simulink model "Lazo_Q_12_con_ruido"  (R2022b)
settings: Solver=ode4  StartTime=0.0  StopTime=0.2  FixedStep=1e-6  RelTol=1e-3
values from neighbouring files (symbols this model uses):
  Delta_v_d_1 = P_Delta_v_d_1*v_d_12    [IP_Lazo_Q_12.m]    (also in LQR_Con_Integral.m = 8; Modal_Integral.m = 8)
  Delta_v_d_2 = P_Delta_v_d_2*v_d_12    [IP_Lazo_Q_12.m]    (also in IP_Lazo_P_2.m = P_Delta_v_d_2*v_d_2)
  I_Delta_v_d_1 = 0.15    [IP_Lazo_Q_12.m]
  I_Delta_v_d_2 = 0.15    [IP_Lazo_Q_12.m]    (also in IP_Lazo_P_2.m)
  Ki_Q = ((3*v_d_12*Kp_Q-2)/(3*v_d_12*tau))    [IP_Lazo_Q_12.m]    (also in Sistema_control_no_lineal_LQR.m = ((3*v_d_1*Kp_Q-2)/(3*v_d_1*tau_Q)); Sistema_control_no_lineal_Modal.m = ((3*v_d_1*Kp_Q-2)/(3*v_d_1*tau_Q)))
  Kp_Q = 1    [IP_Lazo_Q_12.m]    (also in Sistema_control_no_lineal_LQR.m = 0.0002; Sistema_control_no_lineal_Modal.m = 0.0002)
  lim_i_q_1_lower = -576.70686    [IP_Lazo_Q_12.m]    (also in Sistema_control_no_lineal_LQR.m; Sistema_control_no_lineal_Modal.m)
  lim_i_q_1_upper = 393.72177    [IP_Lazo_Q_12.m]    (also in Sistema_control_no_lineal_LQR.m; Sistema_control_no_lineal_Modal.m)
  Q_1_1 = 0    [IP_Lazo_Q_12.m]    (also in Sistema_control_no_lineal_LQR.m; Sistema_control_no_lineal_Modal.m)
  Q_1_2 = -2500    [IP_Lazo_Q_12.m]    (also in Sistema_control_no_lineal_LQR.m = 0; Sistema_control_no_lineal_Modal.m = 0)
  Q_2_1 = -3000    [IP_Lazo_Q_12.m]    (also in Sistema_control_no_lineal_LQR.m = 0; Sistema_control_no_lineal_Modal.m = 0)
  Q_2_2 = 1000    [IP_Lazo_Q_12.m]    (also in Sistema_control_no_lineal_LQR.m = 0; Sistema_control_no_lineal_Modal.m = 0)
  v_d_12 = 100*sqrt(2)    [IP_Lazo_Q_12.m]
  V_R_Q_1 = D_R_Q_1^2    (= 0.0009)    [IP_Lazo_Q_12.m]
  V_R_Q_2 = D_R_Q_2^2    (= 0.0009)    [IP_Lazo_Q_12.m]

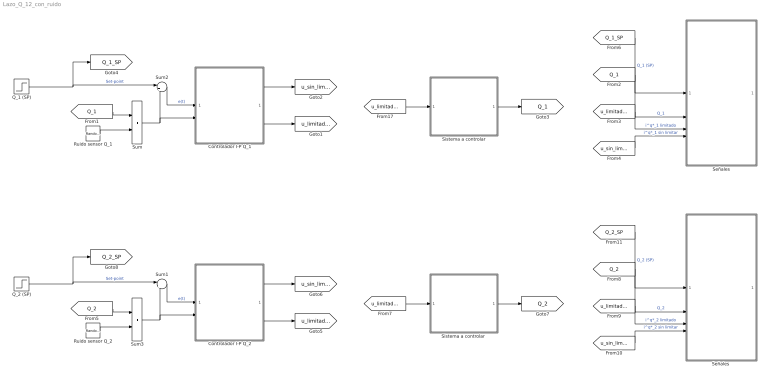
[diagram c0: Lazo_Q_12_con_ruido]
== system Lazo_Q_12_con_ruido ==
  Controlador I-P Q_1 : Subsystem
  Controlador I-P Q_2 : Subsystem
  Q_1 (SP) : Step  Time=0.1  Before=Q_1_1  After=Q_1_2  SampleTime=0
  Q_2 (SP) : Step  Time=0.1  Before=Q_2_1  After=Q_2_2  SampleTime=0
  Ruido sensor Q_1 : RandomNumber  Variance=V_R_Q_1  SampleTime=0.00011
  Ruido sensor Q_2 : RandomNumber  Variance=V_R_Q_2  SampleTime=0.00011
  Señales : Subsystem
  "Señales " : Subsystem
  Sistema a controlar : Subsystem
  "Sistema a controlar " : Subsystem
  Sum : Sum
  Sum1 : Sum  Inputs=|+-
  Sum2 : Sum  Inputs=|+-
  Sum3 : Sum
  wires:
  Q_1 (SP)/1 -> Sum2/1, [Q_1_SP]  "Set-point"
  Sum2/1 -> Controlador I-P Q_1/1(e(t))  "e(t)"
  Controlador I-P Q_1/2(i^q*_1 limitado) -> [u_limitado_1]
  Controlador I-P Q_1/1(i^q*_1 sin limitar) -> [u_sin_limitar_1]
  [u_limitado_1] -> Sistema a controlar/1(i^q*_1 limitado)
  Sistema a controlar/1(Q_1) -> [Q_1]
  [Q_1_SP] -> Señales/1(Q_1 (SP))  "Q_1 (SP)"
  [Q_1] -> Señales/2(Q_1)  "Q_1"
  [u_limitado_1] -> Señales/3(i^q*_1 limitado)  "i^q*_1 limitado"
  [u_sin_limitar_1] -> Señales/4(i^q*_1 sin limitar)  "i^q*_1 sin limitar"
  Sum/1 -> Sum2/2, Controlador I-P Q_1/2(Q_1)
  Sum3/1 -> Sum1/2, Controlador I-P Q_2/2(Q_1)
  [u_sin_limitar_2] -> "Señales "/4(i^q*_2 sin limitar)  "i^q*_2 sin limitar"
  [u_limitado_2] -> "Señales "/3(i^q*_2 limitado)  "i^q*_2 limitado"
  [Q_2] -> "Señales "/2(Q_2)  "Q_2"
  [Q_2_SP] -> "Señales "/1(Q_2 (SP))  "Q_2 (SP)"
  "Sistema a controlar "/1(Q_2) -> [Q_2]
  [u_limitado_2] -> "Sistema a controlar "/1(i^q*_2 limitado)
  Controlador I-P Q_2/1(i^q*_1 sin limitar) -> [u_sin_limitar_2]
  Controlador I-P Q_2/2(i^q*_1 limitado) -> [u_limitado_2]
  Sum1/1 -> Controlador I-P Q_2/1(e(t))  "e(t)"
  Q_2 (SP)/1 -> Sum1/1, [Q_2_SP]  "Set-point"
  [Q_1] -> Sum/1
  Ruido sensor Q_1/1 -> Sum/2
  Ruido sensor Q_2/1 -> Sum3/2
  [Q_2] -> Sum3/1

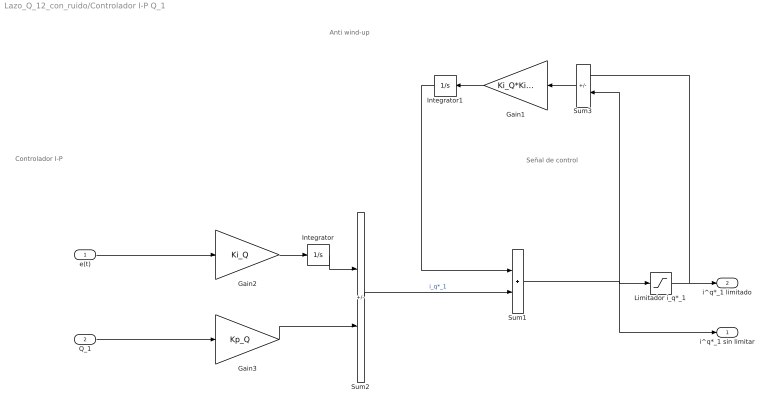
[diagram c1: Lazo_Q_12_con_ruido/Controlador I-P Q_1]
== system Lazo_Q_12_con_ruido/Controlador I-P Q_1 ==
  note: Señal de control
  note: Controlador I-P
  note: Anti wind-up
  e(t) : Inport
  Q_1 : Inport  Port=2
  Gain1 : Gain  Gain=Ki_Q*Ki_Q
  Gain2 : Gain  Gain=Ki_Q
  Gain3 : Gain  Gain=Kp_Q
  Integrator : Integrator
  Integrator1 : Integrator
  Limitador i_q*_1 : Saturate  UpperLimit=lim_i_q_1_upper  LowerLimit=lim_i_q_1_lower
  Sum1 : Sum
  Sum2 : Sum  Inputs=+-
  Sum3 : Sum  Inputs=+-
  i^q*_1 sin limitar : Outport
  i^q*_1 limitado : Outport  Port=2
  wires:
  Limitador i_q*_1/1 -> i^q*_1 limitado/1, Sum3/1
  Sum1/1 -> i^q*_1 sin limitar/1, Limitador i_q*_1/1, Sum3/2
  Sum2/1 -> Sum1/2  "i_q*_1"
  Gain2/1 -> Integrator/1
  Integrator/1 -> Sum2/1
  e(t)/1 -> Gain2/1
  Sum3/1 -> Gain1/1
  Gain1/1 -> Integrator1/1
  Integrator1/1 -> Sum1/1
  Q_1/1 -> Gain3/1
  Gain3/1 -> Sum2/2

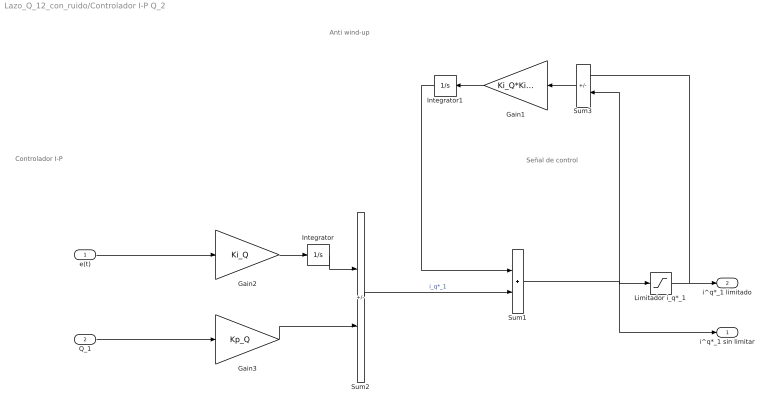
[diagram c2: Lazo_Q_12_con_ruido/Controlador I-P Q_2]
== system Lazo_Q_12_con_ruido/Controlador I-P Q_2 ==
  note: Anti wind-up
  note: Controlador I-P
  note: Señal de control
  e(t) : Inport
  Q_1 : Inport  Port=2
  Gain1 : Gain  Gain=Ki_Q*Ki_Q
  Gain2 : Gain  Gain=Ki_Q
  Gain3 : Gain  Gain=Kp_Q
  Integrator : Integrator
  Integrator1 : Integrator
  Limitador i_q*_1 : Saturate  UpperLimit=lim_i_q_1_upper  LowerLimit=lim_i_q_1_lower
  Sum1 : Sum
  Sum2 : Sum  Inputs=+-
  Sum3 : Sum  Inputs=+-
  i^q*_1 sin limitar : Outport
  i^q*_1 limitado : Outport  Port=2
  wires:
  Gain3/1 -> Sum2/2
  Q_1/1 -> Gain3/1
  Integrator1/1 -> Sum1/1
  Gain1/1 -> Integrator1/1
  Sum3/1 -> Gain1/1
  e(t)/1 -> Gain2/1
  Integrator/1 -> Sum2/1
  Gain2/1 -> Integrator/1
  Sum2/1 -> Sum1/2  "i_q*_1"
  Sum1/1 -> Sum3/2, Limitador i_q*_1/1, i^q*_1 sin limitar/1
  Limitador i_q*_1/1 -> Sum3/1, i^q*_1 limitado/1

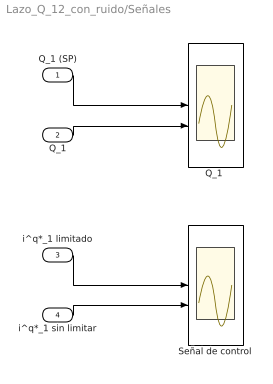
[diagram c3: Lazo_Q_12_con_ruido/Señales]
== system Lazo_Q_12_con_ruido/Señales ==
  Q_1 (SP) : Inport
  Q_1 : Inport  Port=2
  i^q*_1 limitado : Inport  Port=3
  i^q*_1 sin limitar : Inport  Port=4
  "Q_1 " : Scope  NumInputPorts=2
  Señal de control : Scope  NumInputPorts=2
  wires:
  Q_1 (SP)/1 -> "Q_1 "/1
  i^q*_1 sin limitar/1 -> Señal de control/2
  i^q*_1 limitado/1 -> Señal de control/1
  Q_1/1 -> "Q_1 "/2

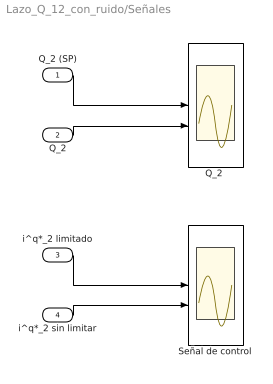
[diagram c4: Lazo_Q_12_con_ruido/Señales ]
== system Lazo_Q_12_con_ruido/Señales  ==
  Q_2 (SP) : Inport
  Q_2 : Inport  Port=2
  i^q*_2 limitado : Inport  Port=3
  i^q*_2 sin limitar : Inport  Port=4
  "Q_2 " : Scope  NumInputPorts=2
  Señal de control : Scope  NumInputPorts=2
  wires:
  Q_2/1 -> "Q_2 "/2
  i^q*_2 limitado/1 -> Señal de control/1
  i^q*_2 sin limitar/1 -> Señal de control/2
  Q_2 (SP)/1 -> "Q_2 "/1

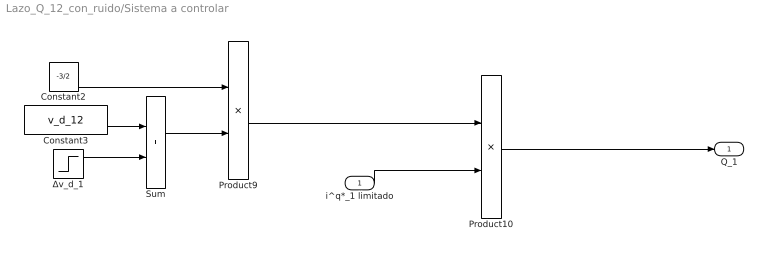
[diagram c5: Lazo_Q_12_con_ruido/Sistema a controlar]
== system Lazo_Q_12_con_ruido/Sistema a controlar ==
  i^q*_1 limitado : Inport
  Constant2 : Constant  Value=-3/2
  Constant3 : Constant  Value=v_d_12
  Product10 : Product
  Product9 : Product
  Sum : Sum
  Δv_d_1 : Step  Time=I_Delta_v_d_1  After=Delta_v_d_1  SampleTime=0
  Q_1 : Outport
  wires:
  Product9/1 -> Product10/1
  i^q*_1 limitado/1 -> Product10/2
  Constant3/1 -> Sum/1
  Constant2/1 -> Product9/1
  Product10/1 -> Q_1/1
  Sum/1 -> Product9/2
  Δv_d_1/1 -> Sum/2

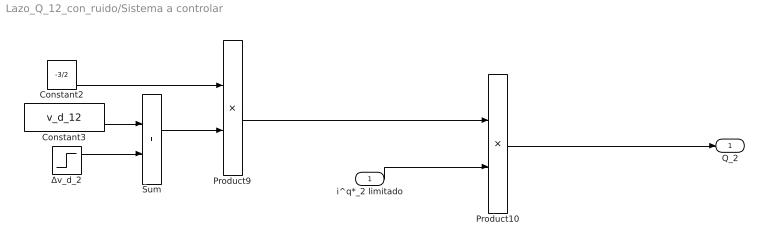
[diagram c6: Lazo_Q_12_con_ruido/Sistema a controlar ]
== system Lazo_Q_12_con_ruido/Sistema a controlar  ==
  i^q*_2 limitado : Inport
  Constant2 : Constant  Value=-3/2
  Constant3 : Constant  Value=v_d_12
  Product10 : Product
  Product9 : Product
  Sum : Sum
  Δv_d_2 : Step  Time=I_Delta_v_d_2  After=Delta_v_d_2  SampleTime=0
  Q_2 : Outport
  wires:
  Product10/1 -> Q_2/1
  i^q*_2 limitado/1 -> Product10/2
  Product9/1 -> Product10/1
  Constant2/1 -> Product9/1
  Δv_d_2/1 -> Sum/2
  Constant3/1 -> Sum/1
  Sum/1 -> Product9/2
